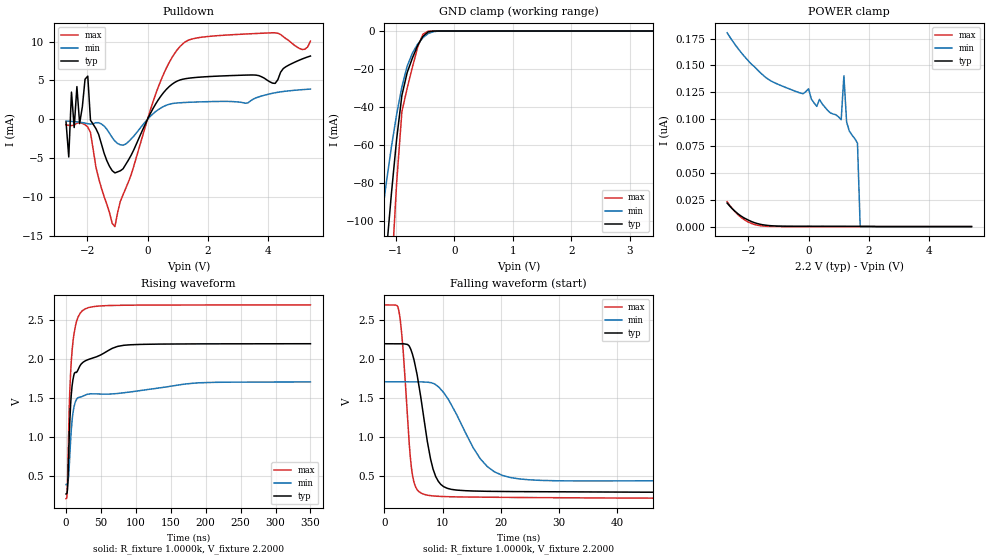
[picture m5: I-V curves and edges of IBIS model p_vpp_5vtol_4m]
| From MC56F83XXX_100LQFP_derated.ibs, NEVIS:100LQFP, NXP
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[Model] p_vpp_5vtol_4m
|   Model p_vpp_5vtol_4m
| Library cells for typ/min/max conditions are connected as defined below:
|  pad_vpp - External Pad
|  ipp_do - Core Input
|  ipp_obe - Output Buffer Enable
|  esd_boost - vdd_s_3v
|  esd_bus - vdd_s_3v
|  ipp_ina_hv - NC
|  ipp_ind - NC
|  ipp_ind_3v - NC
|  tie_3v - vdd_s_3v
|  tie_hi - vdd_s_lv
|  vbuf_3v - vdd_s_3v
|  vdd_bulk_lv - vdd_s_lv
|  vdd_s_3v - vdd_s_3v
|  vdd_s_lv - vdd_s_lv
|  vpp1 - NC
|  vpp2 - NC
|  vss_bulk - vss_s_3v
|  vss_s_3v - vss_s_3v
|  vss_s_lv - vss_s_lv
| All other pins connected to ground
Model_type I/O_open_drain
Polarity   Non-Inverting
Enable   Active-High
Vinl =   0.7700V
Vinh =   1.5400V
Vmeas =  1.1000V
Cref =   25.0000pF
Rref =   0.7000k
Vref =   2.2000V
C_comp   4.4224pF   4.2218pF   4.8247pF
[Temperature Range]   25.0000   0.1250k   -40.0000
[Voltage Range]   2.2000V   1.7100V   2.7000V
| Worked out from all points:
|   slope of the pulldown table from 0 to 0.33 V, typ, clamps not added: 141 ohm
|   GND clamp passes 1 mA (typ) near -0.47 V on its own axis
|   rising waveform, R_fixture 1.0000k, V_fixture 2.2000: 20-80 % time 8.38ns typ, 8.25ns min, 6.9ns max; typ from 0.264 V to 2.2 V
|   falling waveform, R_fixture 1.0000k, V_fixture 2.2000: 20-80 % time 2.55ns typ, 5.89ns min, 1.38ns max; typ from 2.2 V to 0.264 V
[Pulldown]
|Voltage   I(typ)   I(min)   I(max)
-2.7V     -360uA     -220uA     -712uA
-2.61V    -4.841mA   -242uA     -776uA
-2.52V    3.501mA    -265uA     -808uA
-2.43V    -1.056mA   -294uA     -723uA
-2.34V    4.208mA    -328uA     -505uA
-2.25V    -555uA     -370uA     -431uA
-1.98V    5.556mA    -559uA     -987uA
-1.89V    -123uA     -611uA     -1.7mA
-1.08V    -6.893mA   -2.8mA     -13.79mA
360mV     2.527mA    1.256mA    4.189mA
1.17V     5.158mA    2.152mA    9.719mA
5.4V      8.139mA    3.888mA    10.05mA
[GND_clamp]
|Voltage   I(typ)   I(min)   I(max)
-2.7V     -10.22A    -10.77A    -9.929A
-1.35V    -187.5mA   -123.4mA   -295.4mA
-1.26V    -151.8mA   -101.6mA   -237.8mA
-1.17V    -117.6mA   -80.46mA   -182mA
-1.08V    -85.64mA   -61.04mA   -128.9mA
-990mV    -56.78mA   -43.8mA    -79.75mA
-900mV    -33.78mA   -29.29mA   -42.32mA
-810mV    -21.85mA   -18.48mA   -30.07mA
-630mV    -7.548mA   -6.877mA   -8.447mA
-540mV    -2.803mA   -3.492mA   -1.687mA
-450mV    -475.2uA   -1.332mA   -60.39uA
5.4V      0A         0A         0A
[POWER_clamp]
|Voltage   I(typ)   I(min)   I(max)
-2.7V     21.91nA    180.4nA    23.17nA
-1.71V    2.907nA    146.3nA    1.383nA
-450mV    295.2pA    126.1nA    2.244pA
0V        317.8pA    128.3nA    978.9fA
270mV     247.9pA    111.9nA    692.4fA
360mV     247.3pA    118.4nA    692.4fA
1.08V     237pA      99.49nA    525.3fA
1.17V     231.6pA    140.4nA    465.6fA
1.26V     225.8pA    97.42nA    394fA
1.62V     216pA      77.68nA    226.8fA
1.71V     190.3pA    0A         197fA
5.4V      0A         0A         0A
[Ramp]
| variable   typ   min   max
dV/dt_r  0.1642/1.1176n   66.7506m/1.8699n   0.3212/0.8170n
dV/dt_f  0.1640/3.6447n   65.9826m/7.1553n   0.3203/2.0811n
R_load = 50.0000
[Rising Waveform]
R_fixture= 1.0000k
V_fixture= 2.2000
V_fixture_min= 1.7100
V_fixture_max= 2.7000
|time   V(typ)   V(min)   V(max)
0s        264mV      386mV      203.4mV
1.576ns   287.6mV    387.4mV    264.9mV
2.583ns   410.2mV    412.3mV    653.4mV
4.638ns   1.022V     625.3mV    1.406V
6.459ns   1.402V     941.6mV    1.81V
8.342ns   1.634V     1.177V     2.078V
14.9ns    1.831V     1.481V     2.483V
23.01ns   1.949V     1.52V      2.621V
82.88ns   2.179V     1.568V     2.695V
350ns     2.199V     1.707V     2.699V
[Falling Waveform]
R_fixture= 1.0000k
V_fixture= 2.2000
V_fixture_min= 1.7100
V_fixture_max= 2.7000
|time   V(typ)   V(min)   V(max)
0s        2.2V       1.71V      2.7V
2.58ns    2.2V       1.71V      2.585V
3.23ns    2.199V     1.71V      2.11V
4.522ns   2.131V     1.71V      693.3mV
5.621ns   1.801V     1.71V      320.3mV
8.472ns   561.8mV    1.687V     238.3mV
10.79ns   337.5mV    1.505V     229.8mV
17.69ns   298.6mV    616.6mV    222.3mV
26.79ns   292.9mV    439.6mV    217.1mV
350ns     264.3mV    400.4mV    203.5mV
